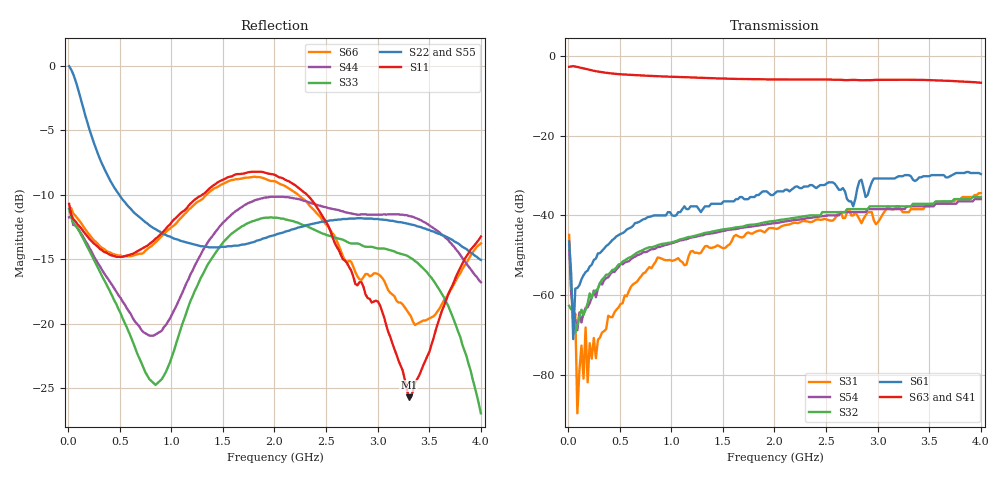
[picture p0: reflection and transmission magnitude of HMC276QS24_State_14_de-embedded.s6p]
! Hittite Microwave Corporation
! 20 Alpha Road
! Chelmsford, MA 01824
! Tel: 978-250-3343
! Fax: 978-250-3373
! Device: HMC276QS24, 0.7-3.0 GHz, GaAS MMIC 4x2 Switch Matrix in 24-lead QSOP package
! Misc: Data was de-embedded to package pins.
!  Port 1 = OP1
!  Port 2 = VL
!  Port 3 = VH
!  Port 4 = HH
!  Port 5 = HL
!  Port 6 = OP2
!  Vdd = +5 V
!  Vctl = 0 V[Logic 0] / +5 V[Logic 1]
!  State 14,  HH to OP1, VH to OP2
!  Control Lines (Logic)
!  HV 1 = 1, Tone 1 = 1
!  HV 2 = 0, Tone 2 = 1
!  Data reformated to new Touchstone file format - Wed Jan 10 15:59:03 2007
# MHz S DB R 50
! 6 Port Network Data
! freq  dbS11  angS11  dbS12  angS12  dbS13  angS13  dbS14  angS14
!  dbS15  angS15  dbS16  angS16
!  dbS21  angS21  dbS22  angS22
!  dbS23  angS23  dbS24  angS24  dbS25  angS25  dbS26  angS26
!  dbS31  angS31  dbS32  angS32  dbS33  angS33  dbS34  angS34
!  dbS35  angS35  dbS36  angS36
!  dbS41  angS41  dbS42  angS42
!  dbS43  angS43  dbS44  angS44  dbS45  angS45  dbS46  angS46
!  dbS51  angS51  dbS52  angS52  dbS53  angS53  dbS54  angS54
!  dbS55  angS55  dbS56  angS56
!  dbS61  angS61  dbS62  angS62
!  dbS63  angS63  dbS64  angS64  dbS65  angS65  dbS66  angS66
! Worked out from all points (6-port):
!   201 points, 10 MHz to 4 GHz, reference 50 ohm
!   strongest paths, dB at 10 MHz, 1.008 GHz, 2.005 GHz, 3.002 GHz, 4 GHz:
!     S63: -2.7, -5.3, -5.9, -6.0, -6.7
!     S41: -2.6, -5.3, -6.1, -6.2, -6.9
!     S61: -46.5, -40.0, -34.4, -30.8, -29.6
!     S32: -62.6, -46.7, -41.4, -37.7, -35.4
!     S54: -47.3, -47.0, -41.9, -38.4, -35.9
!     S31: -44.9, -51.4, -43.3, -41.7, -34.4
!   lowest |S11| = -25.7 dB at 3.302 GHz (marker M1), VSWR 1.11, Z = 54.2 + j3.37 ohm
!   |S11| at or under -10 dB: start of sweep to 1.298 GHz; 2.317 GHz to end of sweep
